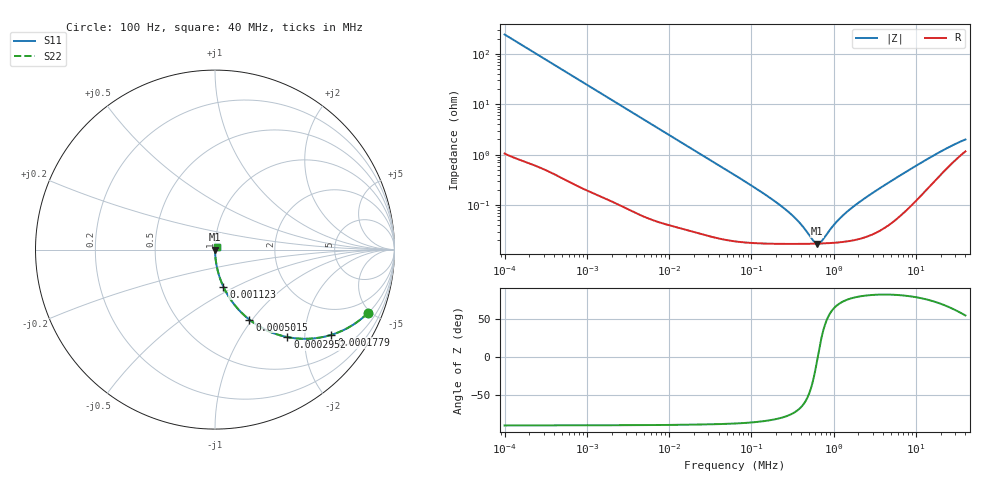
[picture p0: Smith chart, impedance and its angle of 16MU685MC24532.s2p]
!Components F PML CAP
!CONCATENATE F 0.1-40000kHz, at 20deg DC=0V
!Part Number F 16MU685MC24532
!Copyright(C) Rubycon Corporation. 20161129
# MHz S MA R
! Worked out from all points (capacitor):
!   561 points, 100 Hz to 40 MHz, reference 50 ohm
!   read as one part in series: C = 6.58 uF near 104.7 Hz
!   lowest |Z| = 17.3 mohm at 633 kHz (marker M1)
!   series resonance near 641.4 kHz, so ESL is about 9.4 nH
!   S11 on the Smith chart (normalised r, x): 100 Hz: 1.02, -4.83; 177.9 Hz: 1.01, -2.72; 295.2 Hz: 1.01, -1.64; 501.5 Hz: 1.01, -0.97; 1.123 kHz: 1.00, -0.43; 40 MHz: 1.02, +0.03
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0.0001  0.9226 -22.4  0.3818 67.3  0.3818 67.3  0.9226 -22.4
0.0001318391  0.8762 -28.5  0.4779 61.2  0.4779 61.2  0.8762 -28.5
0.0001778656  0.8036 -36.2  0.5909 53.5  0.5909 53.5  0.8036 -36.2
0.0002952384  0.6325 -50.4  0.7706 39.2  0.7706 39.2  0.6325 -50.4
0.0005014845  0.4347 -63.8  0.8975 25.8  0.8975 25.8  0.4347 -63.8
0.0008716573  0.2685 -74.0  0.9612 15.6  0.9612 15.6  0.2685 -74.0
0.001123017  0.2118 -77.3  0.9756 12.2  0.9756 12.2  0.2118 -77.3
0.002573467  0.09464 -84.0  0.9945 5.4  0.9945 5.4  0.09464 -84.0
0.007424854  0.03313 -87.3  0.999 1.9  0.999 1.9  0.03313 -87.3
0.06324555  0.003917 -87.0  0.9998 0.2  0.9998 0.2  0.003917 -87.0
0.1517644  0.001567 -83.6  0.9998 0.1  0.9998 0.1  0.001567 -83.6
0.2637898  0.0008077 -77.8  0.9998 0.0  0.9998 0.0  0.0008077 -77.8
0.381344  0.0004575 -68.1  0.9998 0.0  0.9998 0.0  0.0004575 -68.1
0.5512845  0.0002091 -34.8  0.9998 0.0  0.9998 0.0  0.0002091 -34.8
0.6329915  0.0001731 -4.4  0.9998 0.0  0.9998 0.0  0.0001731 -4.4
0.7102582  0.0001895 23.6  0.9998 -0.0  0.9998 -0.0  0.0001895 23.6
1.0507  0.0004392 65.8  0.9998 -0.0  0.9998 -0.0  0.0004392 65.8
1.484342  0.0007627 75.4  0.9998 -0.0  0.9998 -0.0  0.0007627 75.4
2.407749  0.001378 80.3  0.9998 -0.1  0.9998 -0.1  0.001378 80.3
4.69589  0.002811 81.6  0.9996 -0.2  0.9996 -0.2  0.002811 81.6
19.58601  0.01125 69.5  0.9961 -0.6  0.9961 -0.6  0.01125 69.5
40  0.01998 54.0  0.9884 -0.9  0.9884 -0.9  0.01998 53.9
